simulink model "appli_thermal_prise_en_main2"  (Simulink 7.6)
settings: Solver=ode15s  StartTime=0.0  StopTime=5e3  RelTol=1e-3
StopFcn:
  | close all
  | load temp.mat
  | plot(x(1,:),x(2,:),x(1,:),x(3,:))
  | title('Conduction entre 2 masses thermiques')
  | xlabel('temps')
  | grid
  | gtext('température de la masse thermique 1')
  | gtext('température de la masse thermique 2')
  | delete *.mat
libraries: fl_lib x7, nesl_utility x3

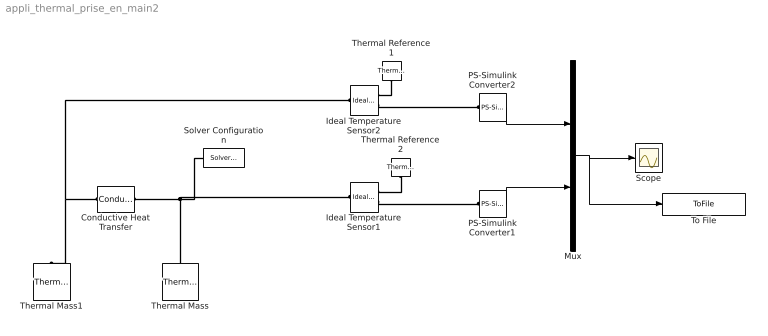
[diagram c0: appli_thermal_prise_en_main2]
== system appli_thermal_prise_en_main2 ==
  Conductive Heat Transfer : fl_lib/Thermal/Thermal Elements/Conductive Heat Transfer  DialogController=NetworkEngine.DynNeDlgSource  SystemSampleTime=-1  area=1e-4 m^2  thickness=0.1 m  th_cond=401 W/(m*K)  Q_Log=off  T_Log=off  LocalVarNames=|Q|T  LocalVarDescs=|Q|T  LocalVarLogging=[0 0]
  Ideal Temperature Sensor1 : fl_lib/Thermal/Thermal Sensors/Ideal Temperature Sensor  DialogController=NetworkEngine.DynNeDlgSource  SystemSampleTime=-1  Qs_Log=off  Ts_Log=off  LocalVarNames=|Qs|Ts  LocalVarDescs=|Qs|Ts  LocalVarLogging=[0 0]
  Ideal Temperature Sensor2 : fl_lib/Thermal/Thermal Sensors/Ideal Temperature Sensor  DialogController=NetworkEngine.DynNeDlgSource  SystemSampleTime=-1  Qs_Log=off  Ts_Log=off  LocalVarNames=|Qs|Ts  LocalVarDescs=|Qs|Ts  LocalVarLogging=[0 0]
  Mux : Mux  Inputs=2
  PS-Simulink Converter1 : nesl_utility/PS-Simulink Converter  DialogController=NetworkEngine.DynNeUtilDlgSource  SystemSampleTime=-1  PhysicalDomain=network_engine_domain  LeftPortType=input  RightPortType=output  SubClassName=ps_output  Unit=1  AffineConversion=off
  PS-Simulink Converter2 : nesl_utility/PS-Simulink Converter  DialogController=NetworkEngine.DynNeUtilDlgSource  SystemSampleTime=-1  PhysicalDomain=network_engine_domain  LeftPortType=input  RightPortType=output  SubClassName=ps_output  Unit=1  AffineConversion=off
  Scope : Scope
  Solver Configuration : nesl_utility/Solver Configuration  DialogController=NetworkEngine.DynNeUtilDlgSource  SystemSampleTime=-1  PhysicalDomain=network_engine_domain  LeftPortType=input  RightPortType=generic  SubClassName=solver  Accelerate=off  Profile=off  ResidualTolerance=1e-9  MaxNonlinIter=12  MaxModeIter=2  DoFixedCost=off  UseLocalSampling=off  DoDC=on  LinearAlgebra=Full  LocalSolverSampleTime=.001  LocalSolverChoice=NE_BACKWARD_EULER_ADVANCER  UseLocalSolver=off
  Thermal Mass : fl_lib/Thermal/Thermal Elements/Thermal Mass  DialogController=NetworkEngine.DynNeDlgSource  SystemSampleTime=-1  mass=0.5 kg  sp_heat=447 J/kg/K  init_temp=273 K  Q_Log=off  LocalVarNames=|Q  LocalVarDescs=|Q  LocalVarLogging=0
  Thermal Mass1 : fl_lib/Thermal/Thermal Elements/Thermal Mass  DialogController=NetworkEngine.DynNeDlgSource  SystemSampleTime=-1  mass=1 kg  sp_heat=447 J/kg/K  init_temp=300 K  Q_Log=off  LocalVarNames=|Q  LocalVarDescs=|Q  LocalVarLogging=0
  Thermal Reference1 : fl_lib/Thermal/Thermal Elements/Thermal Reference  DialogController=NetworkEngine.DynNeDlgSource  SystemSampleTime=-1  Q_Log=off  LocalVarNames=|Q  LocalVarDescs=|Q  LocalVarLogging=0
  Thermal Reference2 : fl_lib/Thermal/Thermal Elements/Thermal Reference  DialogController=NetworkEngine.DynNeDlgSource  SystemSampleTime=-1  Q_Log=off  LocalVarNames=|Q  LocalVarDescs=|Q  LocalVarLogging=0
  To File : ToFile  Filename=temp.mat  MatrixName=x
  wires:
  Mux/1 -> Scope/1, To File/1
  PS-Simulink Converter2/1 -> Mux/1
  PS-Simulink Converter1/1 -> Mux/2
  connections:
  Ideal Temperature Sensor1/RConn2 -- PS-Simulink Converter1/LConn1
  Thermal Reference2/LConn1 -- Ideal Temperature Sensor1/RConn1
  Thermal Mass/LConn1 -- Conductive Heat Transfer/RConn1 -- Ideal Temperature Sensor1/LConn1 -- Solver Configuration/RConn1
  Thermal Reference1/LConn1 -- Ideal Temperature Sensor2/RConn1
  Ideal Temperature Sensor2/RConn2 -- PS-Simulink Converter2/LConn1
  Conductive Heat Transfer/LConn1 -- Thermal Mass1/LConn1 -- Ideal Temperature Sensor2/LConn1
